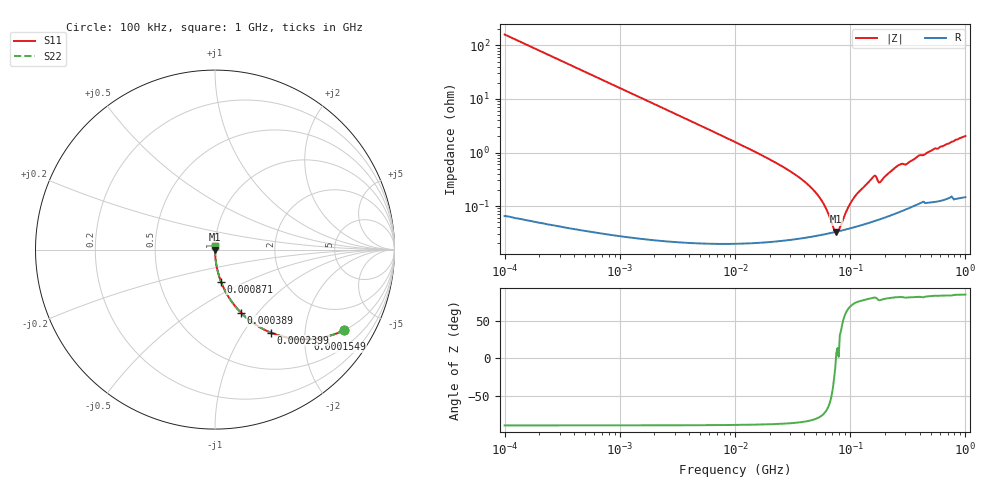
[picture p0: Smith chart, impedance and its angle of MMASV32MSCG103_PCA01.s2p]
! MMASV32MSCG103_PCA01  S-PARAMETER MODEL  ( Standard Model )
! Model Generated by TAIYO YUDEN Corporation (https://www.yuden.co.jp/en/)
! Version 1.0
! TAIYO YUDEN Control No. 250312
! Copyright(c) 2025 TAIYO YUDEN CO.,LTD. All Rights Reserved.
! Product Description (link to TY-COMPAS)
! https://ds.yuden.co.jp/TYCOMPAS/or/detail?pn=MMASV32MSCG103JPCA01&u=M
! Products Name : Multilayer Ceramic Capacitors
! Characteristics :
!  Capacitance : 0.01 [uF] , Rated Voltage : 1000 [V] , TCC : CG / C0G
!  Case Size : 3.2 x 2.5 / 0.126 x 0.098 [mm/inch] , Thickness : 2.5 / 0.098 [mm/inch]
!  (Conditions: Temperature = 25 [degC] , DC Bias Voltage = 0 [V])
! External Node Assignments :
!  1  o---| |---o  2
! GND o---------o GND
! Frequency Range : 0.1MHz  -  1000MHz  [ 401 STEP ]
# MHZ S RI R 50
! Freq[MHz].  S11 Real  S11 Imag  S21 Real  S21 Imag  S12 Real  S12 Imag  S22 Real  S22 Imag
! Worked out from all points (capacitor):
!   401 points, 100 kHz to 1 GHz, reference 50 ohm
!   read as one part in series: C = 9.91 nF near 104.7 kHz
!   lowest |Z| = 33.4 mohm at 75.86 MHz (marker M1)
!   series resonance near 75.21 MHz, so ESL is about 450 pH
!   S11 on the Smith chart (normalised r, x): 100 kHz: 1.00, -3.21; 154.9 kHz: 1.00, -2.07; 239.9 kHz: 1.00, -1.34; 389 kHz: 1.00, -0.83; 871 kHz: 1.00, -0.37; 1 GHz: 1.00, +0.04
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0.1  0.7205 -0.4485  0.2795 0.4485  0.2795 0.4485  0.7205 -0.4485
0.154882  0.5179 -0.4994  0.4821 0.4994  0.4821 0.4994  0.5179 -0.4994
0.239883  0.3094 -0.4619  0.6906 0.4619  0.6906 0.4619  0.3094 -0.4619
0.389045  0.1457 -0.3524  0.8543 0.3524  0.8543 0.3524  0.1457 -0.3524
0.467735  0.1056 -0.3068  0.8944 0.3068  0.8944 0.3068  0.1056 -0.3068
0.870964  0.0331 -0.1781  0.9669 0.1781  0.9669 0.1781  0.0331 -0.1781
2.187762  0.00556 -0.0729  0.9944 0.0729  0.9944 0.0729  0.00556 -0.0729
10  0.000444 -0.0157  0.9996 0.0157  0.9996 0.0157  0.000444 -0.0157
27.54229  0.000252 -0.00503  0.9997 0.00503  0.9997 0.00503  0.000252 -0.00503
46.77351  0.000272 -0.0021  0.9997 0.0021  0.9997 0.0021  0.000272 -0.0021
58.88437  0.000295 -0.00105  0.9997 0.00105  0.9997 0.00105  0.000295 -0.00105
70.79458  0.00032 -0.000263  0.9997 0.000263  0.9997 0.000263  0.00032 -0.000263
75.85776  0.00033 4.47e-05  0.9997 -4.47e-05  0.9997 -4.47e-05  0.00033 4.47e-05
81.28305  0.000342 0.000206  0.9997 -0.000206  0.9997 -0.000206  0.000342 0.000206
97.72372  0.000379 0.000937  0.9996 -0.000937  0.9996 -0.000937  0.000379 0.000937
114.8154  0.000418 0.00165  0.9996 -0.00165  0.9996 -0.00165  0.000418 0.00165
158.4893  0.000525 0.00347  0.9995 -0.00347  0.9995 -0.00347  0.000525 0.00347
181.9701  0.000574 0.00273  0.9994 -0.00273  0.9994 -0.00273  0.000574 0.00273
218.7762  0.00067 0.00417  0.9993 -0.00417  0.9993 -0.00417  0.00067 0.00417
269.1535  0.000809 0.00588  0.9992 -0.00588  0.9992 -0.00588  0.000809 0.00588
309.0295  0.00091 0.00601  0.9991 -0.00601  0.9991 -0.00601  0.00091 0.00601
1000  0.00187 0.0202  0.9981 -0.0202  0.9981 -0.0202  0.00187 0.0202
